(* Logix 5000 DataType export MPE_Input; software revision 33.01 *)

TYPE MPE_Input :   // MPE Input Data Type
STRUCT
   StatusRegQ : DINT[2]; {access Read Only}   // Query status register
   MeasCurrQ : REAL; {access Read Only}   // Query Terminal Current Measurements
   MeasVoltQ : REAL; {access Read Only}   // Query Terminal Voltage Measurements
END_STRUCT
END_TYPE
